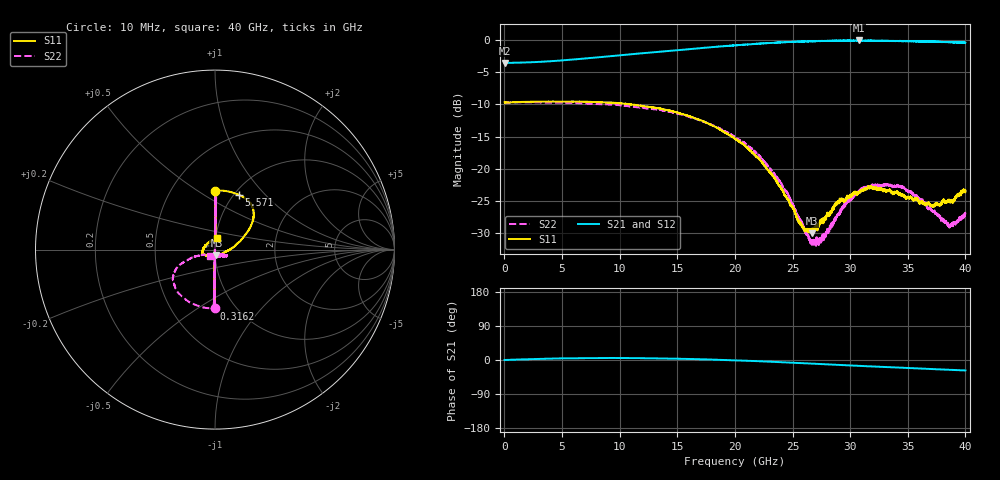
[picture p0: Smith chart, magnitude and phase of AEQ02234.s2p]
! Sonnet Data File
! From: emgraph Version : 16.52
! From Emgraph Data: 1
! Data File Written: 02/28/2018 11:22:32
!< HDATE 02/28/2018 11:20:32
!< MDATE 02/28/2018 11:20:32
# GHZ S MA R 50.00000
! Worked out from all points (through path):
!   6401 points, 10 MHz to 40 GHz, reference 50 ohm
!   highest |S21| = -0.03 dB at 30.77 GHz (marker M1); lowest = -3.5 dB at 16.25 MHz (marker M2)
!   group delay of S21, straight-line fit = 2.32 ps
!   lowest |S11| = -30.0 dB at 26.65 GHz (marker M3), VSWR 1.06, Z = 50.7 - j3.1 ohm
!   |S11| at or under -10 dB: 10.98194 GHz to 10.98258 GHz (640.3 kHz wide, 0.00583 % of centre); 11.02695 GHz to 11.04216 GHz (15.2 MHz wide, 0.138 % of centre); 11.05 GHz to end of sweep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
!   |S22| runs from -32.1 to -9.6 dB; largest |S21 - S12| = 0.0068
!   S11 on the Smith chart (normalised r, x): 10 MHz: 0.80, +0.59; 316.2 MHz: 0.79, -0.58; 5.571 GHz: 1.06, +0.72; 40 GHz: 1.01, +0.14
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0.01  0.329 90.0  0.6669 0.0  0.6652 0.0  0.3241 -90.3
0.01624844  0.3278 90.1  0.6663 0.1  0.6682 0.1  0.3263 -90.0
0.1412172  0.3281 89.4  0.667 0.1  0.6669 0.1  0.3263 -90.6
0.2724344  0.3283 88.9  0.6673 0.3  0.6674 0.3  0.3266 -91.2
0.3161734  0.3282 -91.3  0.6667 0.3  0.6668 0.3  0.3263 88.6
0.6723344  0.3293 87.1  0.6677 0.7  0.6681 0.7  0.3271 -93.0
5.571109  0.3331 66.1  0.7034 4.6  0.7033 4.6  0.3255 -115.7
6.677083  0.3322 62.0  0.7175 5.0  0.7172 5.0  0.3225 -120.3
13.34417  0.2952 43.1  0.8125 4.1  0.8122 4.1  0.2883 -144.7
20.005  0.1711 23.1  0.9133 -0.9  0.9135 -0.9  0.1764 -158.9
23.71032  0.07681 -2.0  0.9602 -5.3  0.9592 -5.3  0.08393 -157.6
25.90352  0.03457 -49.4  0.9786 -8.4  0.9789 -8.5  0.03635 -133.7
26.65334  0.03146 -75.8  0.9845 -9.5  0.9814 -9.5  0.02717 -101.2
26.67208  0.03268 -77.4  0.9833 -9.6  0.9816 -9.6  0.02555 -99.5
27.63434  0.04081 -109.0  0.985 -10.9  0.9873 -11.1  0.02982 -65.8
29.04024  0.05514 -139.4  0.9903 -12.9  0.9917 -13.0  0.04361 -36.6
30.77106  0.06462 -156.5  0.9967 -15.4  0.9967 -15.4  0.06643 -27.0
33.33917  0.06772 -178.1  0.9905 -18.9  0.9905 -19.0  0.0736 -29.1
34.6201  0.06128 169.3  0.9813 -20.6  0.9817 -20.6  0.07054 -33.8
37.13197  0.05093 126.7  0.9785 -23.9  0.978 -24.0  0.04665 -52.9
38.61285  0.05602 99.5  0.9662 -25.9  0.969 -25.8  0.03475 -88.6
40  0.06745 80.5  0.9579 -27.5  0.9551 -27.5  0.04502 -124.8
